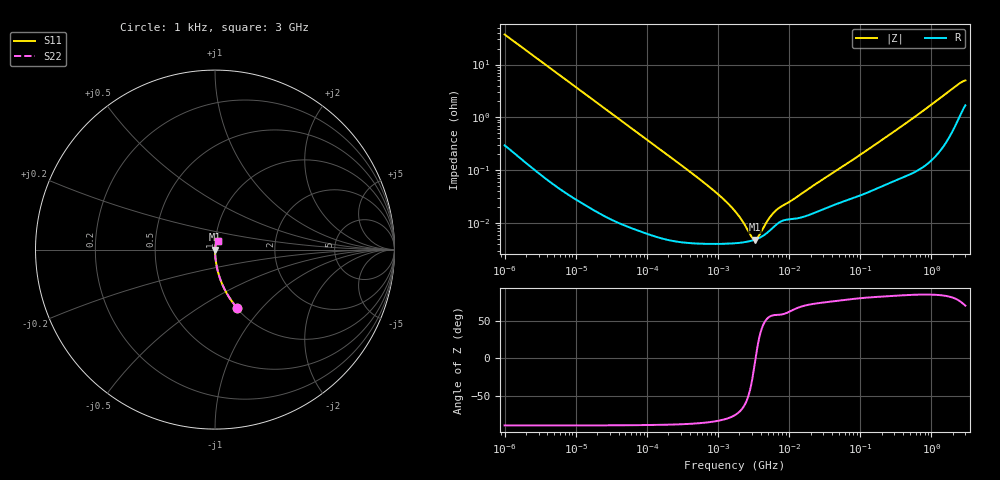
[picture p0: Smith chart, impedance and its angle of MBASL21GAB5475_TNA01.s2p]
! MBASL21GAB5475_TNA01  S-PARAMETER MODEL  ( Standard Model )
! Model Generated by TAIYO YUDEN Corporation (http://www.ty-top.com)
! Version 1.0
! TAIYO YUDEN Control No. 220601
! Copyright(c) 2012 TAIYO YUDEN CO.,LTD. All Rights Reserved.
! Product Description (link to TY-COMPAS)
! https://ds.yuden.co.jp/TYCOMPAS/or/detail?pn=MBASL21GAB5475KTNA01&u=M
! Products Name : Multilayer Ceramic Capacitors
! Characteristics :
!  Capacitance : 4.7 [uF] , Rated Voltage : 10 [V] , TCC : X5R
!  Case Size : 2.0 x 1.25 / 0.079 x 0.049 [mm/inch] , Thickness : 1.25 / 0.049 [mm/inch]
!  (Conditions: Temperature = 25 [degC] , DC Bias Voltage = 0 [V])
! External Node Assignments :
!  1  o---| |---o  2
! GND o---------o GND
! Frequency Range : 1kHz  -  3GHz  [ 401 STEP ]
# MHZ S RI R 50
! Freq[MHz].  S11 Real  S11 Imag  S21 Real  S21 Imag  S12 Real  S12 Imag  S22 Real  S22 Imag
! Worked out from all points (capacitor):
!   401 points, 1 kHz to 3 GHz, reference 50 ohm
!   read as one part in series: C = 4.28 uF near 1.077 kHz
!   lowest |Z| = 4.85 mohm at 3.265 MHz (marker M1)
!   series resonance near 3.372 MHz, so ESL is about 520 pH
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0.001  0.1232 -0.3247  0.8768 0.3247  0.8768 0.3247  0.1232 -0.3247
0.001685  0.048 -0.21  0.952 0.21  0.952 0.21  0.048 -0.21
0.00306  0.0155 -0.12  0.9845 0.12  0.9845 0.12  0.0155 -0.12
0.005768  0.00464 -0.0646  0.9954 0.0646  0.9954 0.0646  0.00464 -0.0646
0.01216  0.00119 -0.0308  0.9988 0.0308  0.9988 0.0308  0.00119 -0.0308
0.147855  5.92e-05 -0.00256  0.9999 0.00256  0.9999 0.00256  5.92e-05 -0.00256
0.791611  4.03e-05 -0.000455  1 0.000455  1 0.000455  4.03e-05 -0.000455
1.238299  4.04e-05 -0.000267  1 0.000267  1 0.000267  4.04e-05 -0.000267
1.732051  4.13e-05 -0.000162  1 0.000162  1 0.000162  4.13e-05 -0.000162
2.166294  4.25e-05 -0.000104  1 0.000104  1 0.000104  4.25e-05 -0.000104
2.334012  4.31e-05 -8.55e-05  1 8.55e-05  1 8.55e-05  4.31e-05 -8.55e-05
3.264662  4.79e-05 -7.36e-06  1 7.36e-06  1 7.36e-06  4.79e-05 -7.36e-06
4.399271  5.84e-05 6.1e-05  0.9999 -6.1e-05  0.9999 -6.1e-05  5.84e-05 6.1e-05
4.739869  6.27e-05 7.82e-05  0.9999 -7.82e-05  0.9999 -7.82e-05  6.27e-05 7.82e-05
5.928204  8.17e-05 0.000128  0.9999 -0.000128  0.9999 -0.000128  8.17e-05 0.000128
6.881678  9.73e-05 0.000156  0.9999 -0.000156  0.9999 -0.000156  9.73e-05 0.000156
21.06097  0.000149 0.00047  0.9999 -0.00047  0.9999 -0.00047  0.000149 0.00047
256.0921  0.000589 0.00463  0.9994 -0.00463  0.9994 -0.00463  0.000589 0.00463
700.8126  0.00121 0.0122  0.9988 -0.0122  0.9988 -0.0122  0.00121 0.0122
2226.275  0.00892 0.0384  0.9911 -0.0384  0.9911 -0.0384  0.00892 0.0384
2682.519  0.0146 0.044  0.9854 -0.044  0.9854 -0.044  0.0146 0.044
3000  0.0187 0.0455  0.9813 -0.0455  0.9813 -0.0455  0.0187 0.0455
